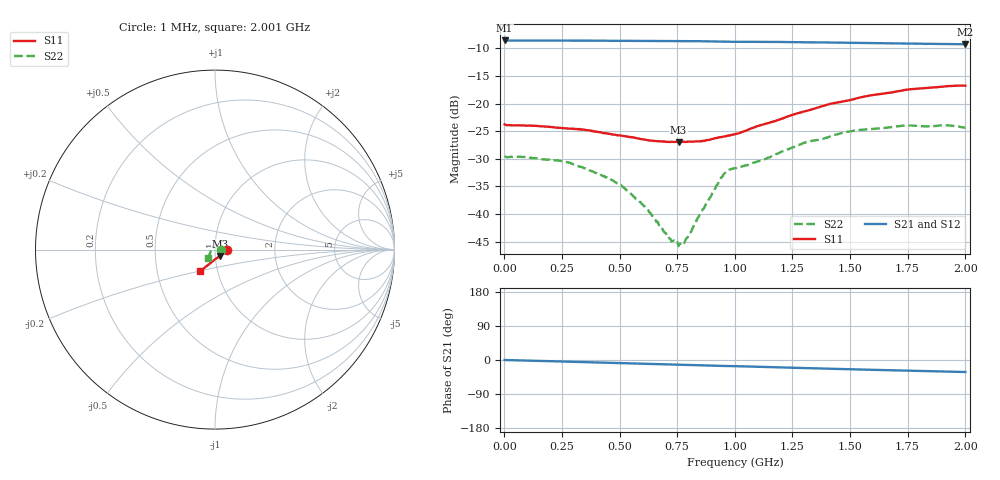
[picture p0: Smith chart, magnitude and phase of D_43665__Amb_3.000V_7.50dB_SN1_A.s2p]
! device id: 43665_
! dir: \\malibu\benchdata\1_engineers\tn_data\43665_75ohm\new\sparar\43665_\amb\3p000v\7p50db
! Serial: 1
! Insertion: A
! Temp: Amb
! VDD: 3.000V
! Attenuation Step: 7.50dB
! IDD: 1.452888e+00mA
! FILE NAME
! DATE 03-27-2009 08:35:12
! CORRECTED  DATA
#  Hz  S  RI  R  75
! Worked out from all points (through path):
!   401 points, 1 MHz to 2.001 GHz, reference 75 ohm
!   highest |S21| = -8.58 dB at 1 MHz (marker M1); lowest = -9.3 dB at 2.001 GHz (marker M2)
!   group delay of S21, straight-line fit = 44.8 ps
!   lowest |S11| = -27.0 dB at 756 MHz (marker M3), VSWR 1.09, Z = 79.1 - j5.52 ohm
!   |S11| at or under -10 dB: start of sweep to end of sweep
!   |S22| runs from -45.8 to -23.9 dB; largest |S21 - S12| = 0.0014
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1000000  0.0649 -0.000964  0.3722 -0.00057  0.3724 -0.000511  0.0335 -0.000251
2.36e8  0.06 -0.00771  0.3704 -0.0242  0.3706 -0.0243  0.0292 0.00859
3.36e8  0.0573 -0.0119  0.3692 -0.0346  0.3693 -0.0347  0.024 0.0114
4.56e8  0.0505 -0.0164  0.3673 -0.0471  0.3675 -0.0472  0.0174 0.0114
5.16e8  0.0467 -0.0201  0.366 -0.0534  0.366 -0.0535  0.0138 0.0108
6.11e8  0.0397 -0.0254  0.3634 -0.063  0.3634 -0.0631  0.00645 0.00983
6.71e8  0.035 -0.0292  0.362 -0.0692  0.3619 -0.0693  0.00294 0.00739
7.16e8  0.0315 -0.0319  0.3606 -0.074  0.3606 -0.074  0.000386 0.00604
7.56e8  0.028 -0.0348  0.3593 -0.0783  0.3594 -0.0783  -0.0027 0.00436
7.71e8  0.0269 -0.036  0.3587 -0.0799  0.3587 -0.0799  -0.00398 0.0037
7.91e8  0.0251 -0.0373  0.3579 -0.0821  0.358 -0.0821  -0.00558 0.00238
8.61e8  0.0178 -0.0425  0.3549 -0.0897  0.3548 -0.0896  -0.0105 -0.00363
9.51e8  0.00805 -0.0495  0.3493 -0.0976  0.3495 -0.0974  -0.0207 -0.00961
9.71e8  0.00648 -0.051  0.3487 -0.0988  0.3488 -0.0986  -0.0233 -0.00895
1.001e9  0.00325 -0.0527  0.3481 -0.1011  0.3483 -0.1011  -0.0245 -0.00876
1.126e9  -0.0108 -0.064  0.3434 -0.1135  0.3437 -0.1134  -0.0267 -0.0165
1.336e9  -0.0343 -0.0818  0.3323 -0.1327  0.3327 -0.1328  -0.0332 -0.032
1.511e9  -0.0526 -0.0953  0.3218 -0.1473  0.3223 -0.1476  -0.0372 -0.0426
1.671e9  -0.0662 -0.1065  0.3124 -0.1593  0.3124 -0.16  -0.0385 -0.0472
1.746e9  -0.0716 -0.1127  0.3078 -0.1646  0.3079 -0.1655  -0.0388 -0.0501
1.916e9  -0.0804 -0.1184  0.2977 -0.1755  0.2975 -0.1756  -0.0399 -0.0495
2.001e9  -0.0822 -0.1195  0.2928 -0.1806  0.2917 -0.1815  -0.0381 -0.0469
